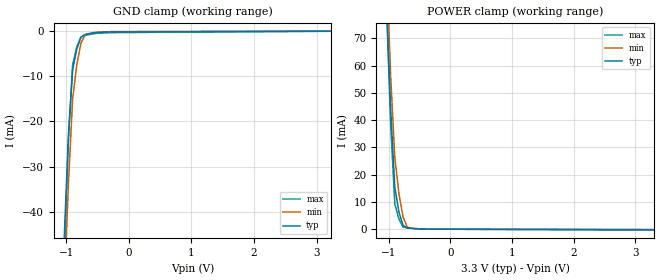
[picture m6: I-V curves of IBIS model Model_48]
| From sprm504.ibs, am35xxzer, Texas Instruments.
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| Model based on original model for IC1833DVTPBFHP18LL_7LM
|   Sub model _7LM_!PI_PUPDSEL_3P3
[model]   Model_48
|[Description]  3.3V-INPUT-PU-X
|[Input Load]   PU
|[Output Drive]
|Voltage   3.3V
|Mode   INPUT
Model_type   Input
Polarity   Non-Inverting
Vinl =  0.8V
Vinh =  2V
C_comp   1.012258p   0.8890016p   1.091755p
[Model Spec]
Vinl   0.8V   0.8V   0.8V
Vinh   2V   2V   2V
[Temperature Range]   25   125   -40
[Voltage Range]   3.3   2.97   3.63
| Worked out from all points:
|   GND clamp passes 1 mA (typ) near -0.73 V on its own axis
|   POWER clamp passes 1 mA (typ) near -0.74 V on its own axis
[POWER_clamp]
-3.3V     2.37A      2.826A     2.542A
-1.033V   82.45mA    94.83mA    80.46mA
-966.7mV  43.63mA    55.94mA    38.29mA
-900mV    15.26mA    26.28mA    9.247mA
-833.3mV  6.359mA    13.02mA    3.717mA
-766.7mV  1.418mA    4.545mA    810uA
-700mV    434uA      841.5uA    527uA
-500mV    113.3uA    72.23uA    139.6uA
3.3V      -177.5uA   -119.9uA   -277.3uA
[GND_clamp]
-3.3V     -1.792A    -1.668A    -2.631A
-1.033V   -45.64mA   -57.79mA   -50.41mA
-966.7mV  -22.95mA   -33.88mA   -24.23mA
-900mV    -8.665mA   -15.12mA   -7.531mA
-833.3mV  -3.992mA   -7.443mA   -3.487mA
-766.7mV  -1.349mA   -2.681mA   -1.294mA
-700mV    -737.2uA   -832.6uA   -950.7uA
-566.7mV  -426.4uA   -322.3uA   -590.6uA
-300mV    -206.6uA   -111.9uA   -344.2uA
3.233V    -3.53uA    8.883uA    -32.96uA
